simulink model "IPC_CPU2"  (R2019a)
settings: Solver=FixedStepDiscrete  StartTime=0.0  StopTime=Inf  RelTol=1e-3  EnableMultiTasking=on
libraries: c2837xDlib x1

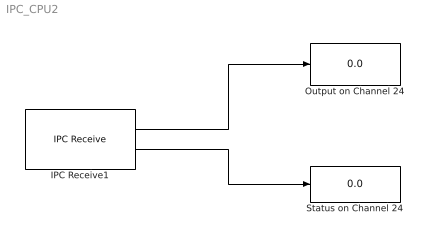
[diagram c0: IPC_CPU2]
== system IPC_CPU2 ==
  IPC Receive1 : c2837xDlib/IPC Receive  SelectChannel=24  DataType=uint32  DataLength=1  EnableBlocking=off  SampleTime=0.5
  Output on Channel 24 : Display
  Status on Channel 24 : Display
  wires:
  IPC Receive1/2 -> Status on Channel 24/1
  IPC Receive1/1 -> Output on Channel 24/1
